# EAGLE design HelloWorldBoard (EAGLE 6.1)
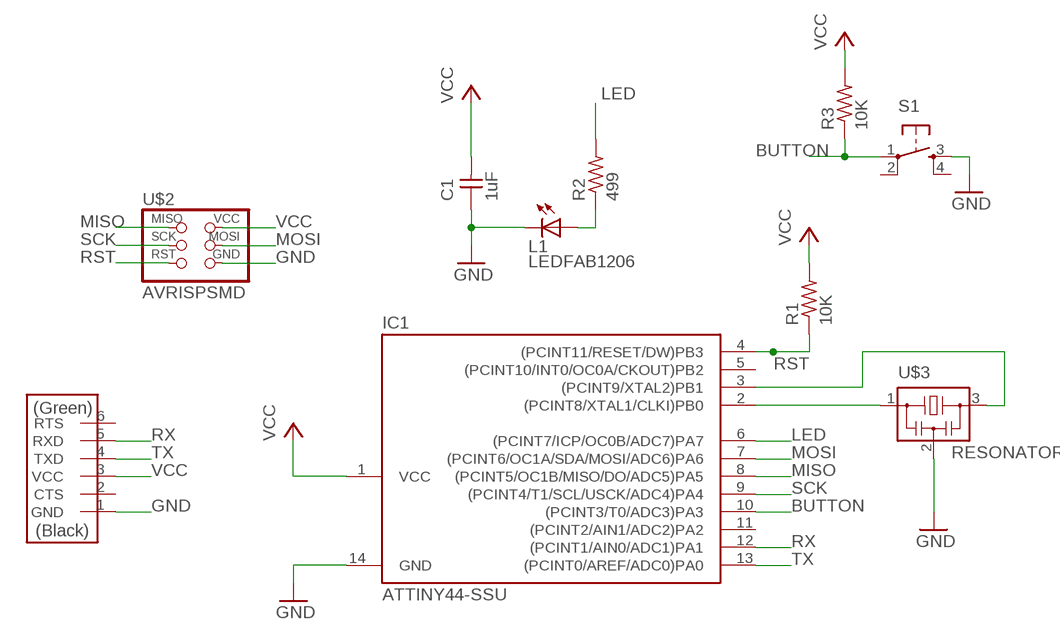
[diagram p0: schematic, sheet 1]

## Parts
C1  1uF  CAP-UNPOLARIZED  [C1206]
IC1  ATTINY44-SSU  [SOIC14]
L1  LEDFAB1206  [LED1206FAB]
R1  10K  RES-US1206FAB  [R1206FAB]
R2  499  RES-US1206FAB  [R1206FAB]
R3  10K  RES-US1206FAB  [R1206FAB]
S1  6MM_SWITCH6MM_SWITCH  [6MM_SWITCH]
U$1  FTDI-SMD-HEADER  [1X06SMD]
U$2  AVRISPSMD  [2X03SMD]
U$3  RESONATOR  [EFOBM]

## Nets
BUTTON: IC1.10((PCINT3/T0/ADC3)PA3) R3.1 S1.1(P)
GND: C1.1 IC1.14(GND) L1.2(C) S1.3(S) U$1.1(GND) U$2.6(GND) U$3.2
LED: IC1.6((PCINT7/ICP/OC0B/ADC7)PA7) R2.2
MISO: IC1.8((PCINT5/OC1B/MISO/DO/ADC5)PA5) U$2.1(MISO)
MOSI: IC1.7((PCINT6/OC1A/SDA/MOSI/ADC6)PA6) U$2.4(MOSI)
N$5: IC1.2((PCINT8/XTAL1/CLKI)PB0) U$3.1
N$6: IC1.3((PCINT9/XTAL2)PB1) U$3.3
R2: L1.1(A) R2.1
RST: IC1.4((PCINT11/RESET/DW)PB3) R1.1 U$2.5(RST)
RX: IC1.12((PCINT1/AIN0/ADC1)PA1) U$1.5(RXD)
SCK: IC1.9((PCINT4/T1/SCL/USCK/ADC4)PA4) U$2.3(SCK)
TX: IC1.13((PCINT0/AREF/ADC0)PA0) U$1.4(TXD)
VCC: C1.2 IC1.1(VCC) R1.2 R3.2 U$1.3(VCC) U$2.2(VCC)
Unconnected: IC1.5((PCINT10/INT0/OC0A/CKOUT)PB2) IC1.11((PCINT2/AIN1/ADC2)PA2) S1.2(P1) S1.4(S1) U$1.2(CTS) U$1.6(RTS)

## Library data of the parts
C1 = fab:CAP-UNPOLARIZED
IC1 = fab:ATTINY44
L1 = fab:LED: LED
R1-R3 = fab:RES-US: Resistor (US Symbol)
S1 = fab:6MM_SWITCH: OMRON SWITCH
U$1 = fab:FTDI-SMD-HEADER
U$2 = fab:AVRISP
U$3 = fab:RESONATOR

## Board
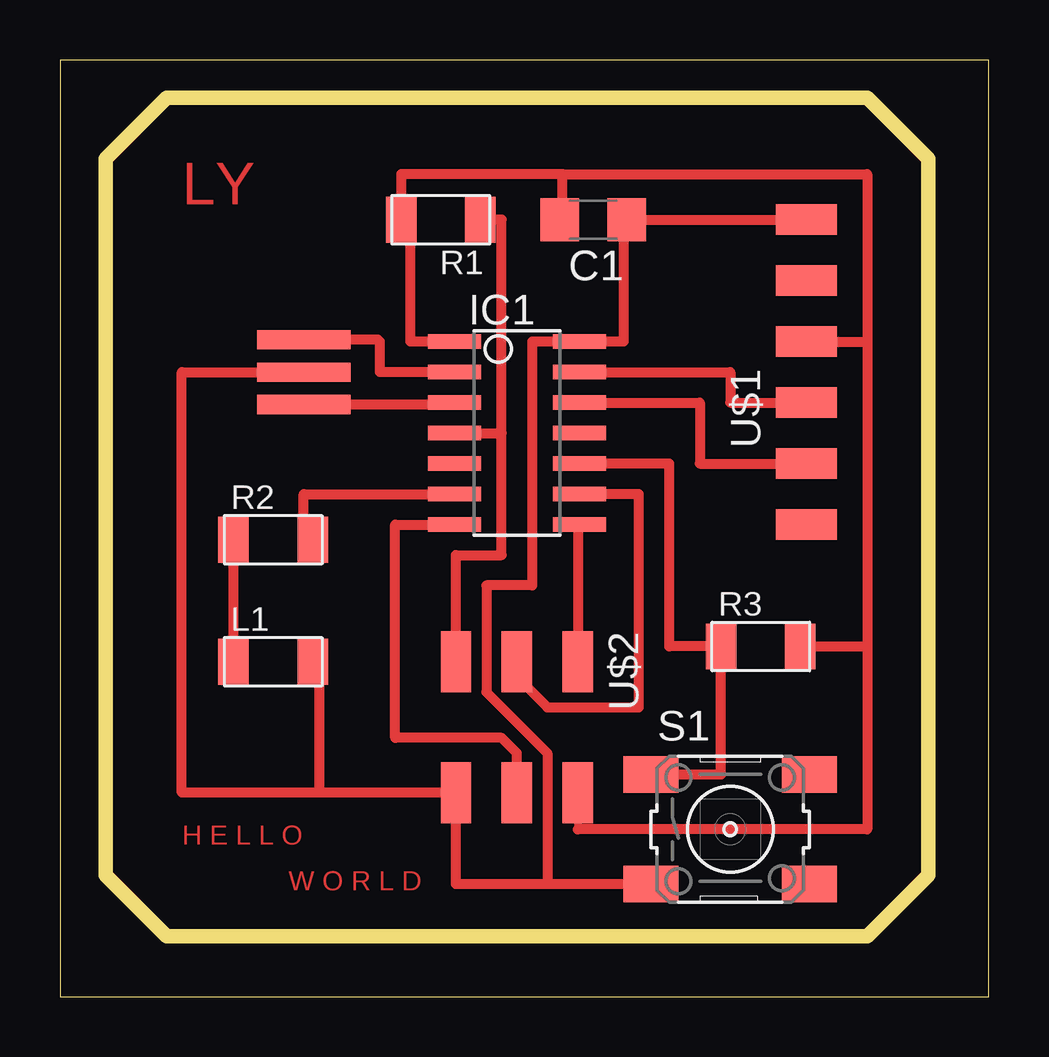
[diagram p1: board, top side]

Size 38.72 x 39.04 mm. Coordinates in mm from the lower left corner, seen from the top.
Outline: 0,0 38.72,0 38.72,39.04 0,39.04 0,0
Outline: 4.45,37.47 1.91,34.92 1.91,5.08 4.45,2.54 33.66,2.54 36.2,5.08 36.2,34.92 33.66,37.47 4.45,37.47
Copper layers (1*16): Top 0.035mm / dielectric 1.5mm / Bottom 0.035mm
Design rules "default": minimum track width 10mil, minimum drill 24mil, track to track 8mil, track to pad 8mil, pad to pad 8mil, via to via 8mil, smd to smd 8mil, copper to edge 40mil, drill to drill 8mil, minimum pad ring 10mil, minimum via ring 8mil, stop-mask expansion 4mil, vias tented up to drill 0mil, thermal gap 10mil

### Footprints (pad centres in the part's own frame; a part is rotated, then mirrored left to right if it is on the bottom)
C1206 = smd 1.6 x 1.8: 1 -1.4,0; 2 1.4,0
SOIC14 = smd 0.61 x 2.21: 1 -3.81,-2.603; 2 -2.54,-2.603; 3 -1.27,-2.603; 4 0,-2.603; 5 1.27,-2.603; 6 2.54,-2.603; 7 3.81,-2.603; 8 3.81,2.603; 9 2.54,2.603; 10 1.27,2.603; 11 0,2.603; 12 -1.27,2.603; 13 -2.54,2.603; 14 -3.81,2.603
LED1206FAB = smd 1.27 x 1.905: 1 -1.651,0; 2 1.651,0
R1206FAB = smd 1.27 x 1.905: 1 -1.651,0; 2 1.651,0
6MM_SWITCH = smd 2.286 x 1.524: 1 -3.302,2.286; 2 3.302,2.286; 3 -3.302,-2.286; 4 3.302,-2.286
1X06SMD = smd 2.54 x 1.27: 1 0,6.35; 2 0,3.81; 3 0,1.27; 4 0,-1.27; 5 0,-3.81; 6 0,-6.35
2X03SMD = smd 2.54 x 1.27: 1 -2.54,2.54; 2 2.92,2.54; 3 -2.54,0; 4 2.92,0; 5 -2.54,-2.54; 6 2.92,-2.54
EFOBM = smd 0.8 x 3.9: 1 -1.35,0; 2 0,0; 3 1.35,0

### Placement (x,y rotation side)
C1  22.23,32.38 180 top
IC1  19.05,23.5 270 top
L1  8.89,13.97 0 top
R1  15.88,32.38 180 top
R2  8.89,19.05 0 top
R3  29.21,14.61 0 top
S1  27.94,6.99 0 top
U$1  31.11,26.04 0 top
U$2  19.05,11.43 270 top
U$3  10.16,26.04 270 top

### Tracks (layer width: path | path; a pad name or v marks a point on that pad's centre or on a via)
BUTTON
  Top 0.406: S1.1 27.56,9.27 R3.1 25.4,14.61 25.4,22.23 IC1.10
GND
  Top 0.305: C1.1 23.5,32.38 | L1.2 10.79,13.97
  Top 0.406: 23.5,32.38 23.5,27.3 IC1.14 19.68,27.3 19.68,17.14 17.78,17.14 17.78,12.7 20.32,10.16 20.32,4.7 | C1.1 U$1.1 | S1.3 20.32,4.7 | 20.32,4.7 16.51,4.7 U$2.6 10.79,8.51 | 10.79,8.51 5.08,8.51 5.08,26.04 U$3.2 | 10.79,13.97 10.79,8.51
LED
  Top 0.305: R2.2 10.16,19.05
  Top 0.406: 10.16,19.05 10.16,20.95 IC1.6
MISO
  Top 0.305: IC1.8 21.59,19.68
  Top 0.406: 21.59,19.68 U$2.1
MOSI
  Top 0.406: U$2.4 19.05,10.16 18.41,10.79 13.97,10.79 13.97,19.68 IC1.7
N$5
  Top 0.305: 13.34,27.3 13.26,27.39
  Top 0.406: IC1.2 13.34,26.04 13.34,27.3 | 13.26,27.39 U$3.1
N$6
  Top 0.305: IC1.3 16.37,24.68
  Top 0.406: 16.37,24.68 U$3.3
R2
  Top 0.406: L1.1 R2.1
RST
  Top 0.406: U$2.5 16.51,18.41 18.41,18.41 18.41,23.5 | IC1.4 18.41,23.5 | 18.41,23.5 18.41,32.38 R1.1
RX
  Top 0.406: IC1.12 26.67,24.77 26.67,22.23 U$1.5
SCK
  Top 0.305: U$2.3 19.05,13.34
  Top 0.406: 19.05,13.34 20.32,12.06 24.13,12.06 24.13,20.95 IC1.9
TX
  Top 0.406: IC1.13 27.94,26.04 27.94,24.77 U$1.4
VCC
  Top 0.305: 21.59,6.99 U$2.2 | 14.61,32.38 R1.2 | C1.2 20.95,32.38 20.95,32.52 C1.2
  Top 0.406: 20.95,34.29 33.66,34.29 33.66,27.3 | U$1.3 33.66,27.3 | 33.66,27.3 33.66,14.61 | R3.2 33.66,14.61 | 33.66,14.61 33.66,6.99 21.59,6.99 | IC1.1 14.61,27.3 14.61,32.38 | 20.95,32.52 20.95,34.29 | 20.95,34.29 14.22,34.29 R1.2

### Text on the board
Top: LY | H E L L O | W O R L D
